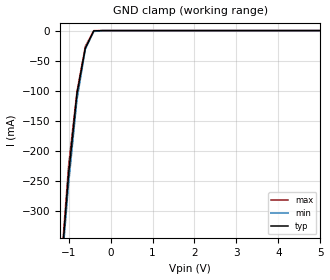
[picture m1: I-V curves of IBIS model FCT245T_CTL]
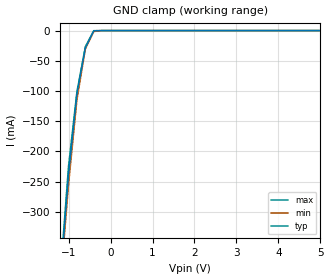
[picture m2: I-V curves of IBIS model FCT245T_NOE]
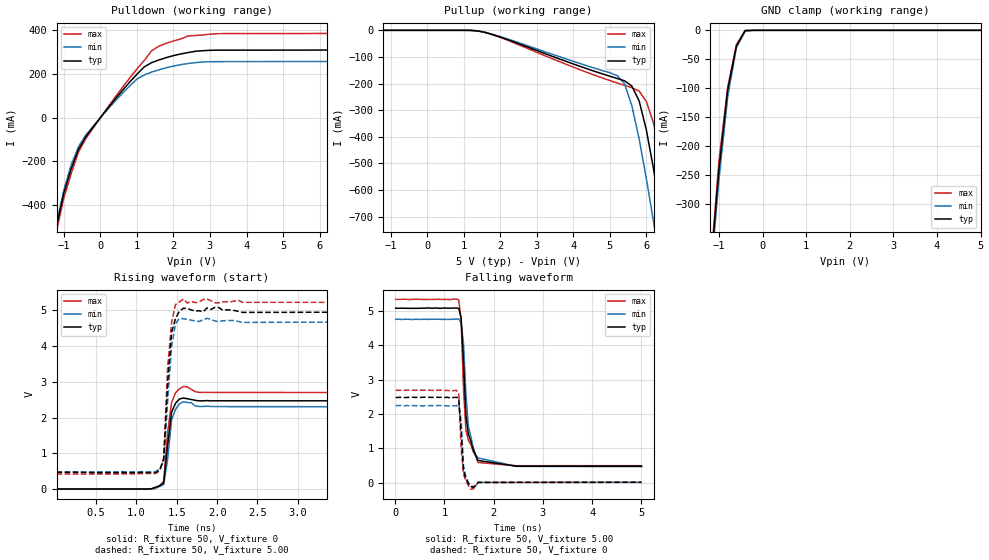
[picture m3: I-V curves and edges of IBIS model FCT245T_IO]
|   TEXAS INSTRUMENTS INCORPORATED
|   Standard Linear and Logic
|   IBIS Model of CY74FCT245T
|   8-BIT TRANSCEIVERS WITH 3-STATE OUTPUTS
|   DIP 20-pin (P), QSOP 20-pin (Q), SOIC 20-pin (SO)
[IBIS Ver]   3.1
[Comment Char]  |_char
[File Name]   cy74fct245t.ibs
[File Rev]   1.1
[Date]   June 4, 2004
[Source]   File originated at Texas Instruments, Inc.
[Notes]   The following is a sample IBIS file for the FCT245T.
   - FILE REV HISTORY
   - 1.1 Release IBIS file on 06/08/04
   - All test data contained in this file are derived from
   actual measurements.
   - Power clamp data deleted as there is no power-clamp diode.
   - The measurement used P package.
[Disclaimer] Property of Texas Instruments Incorporated.  Unauthorized
   reproduction and/or distribution is strictly prohibited.
   This product is protected under copyright law.
   Created 2000, (C) Copyright 2000, Texas Instruments Inc.,
   All Rights Reserved.
   UNLESS THERE IS A SIGNED, WRITTEN AGREEMENT TO THE
   CONTRARY, TEXAS INSTRUMENTS () IS PROVIDING THE IBIS
   MODELS  AND WITHOUT ANY WARRANTY, EXPRESSED OR
   IMPLIED.  TI assumes no liability for:
   1) the accuracy of the IBIS models provided to your
   company;
   2) the proper functioning of these IBIS Models in your
   design or for any resulting applications; or
   3) infringement of patents, copyrights or intellectual
   property rights resulting from your use of these IBIS
   models.
   TI provides IBIS Models as a service to our customers.
   You and your company shall not distribute, sell or give
   these models to anyone else without prior written
   permission from TI.
   TI reserves the right to make changes to our products or
   to discontinue any semiconductor product or service
   without notice, and advises our customers to obtain the
   latest version of relevant information to verify, before
   placing orders, that the information being relied on is
   current.
   Please be aware that your receipt and use of the IBIS
   information provided shall serve as acceptance of these
   terms and conditions.  If you do not accept these terms,
   you should return or destroy the IBIS models and any
   other accompanying information immediately.
|   Component FCT245T_P
[Component]   FCT245T_P
[Manufacturer]  Texas Instruments, Inc.
[Package]
|   typ   min   max
R_pkg   0.043   0.038   0.05
L_pkg   7.384nH   4.68nH   10.321nH
C_pkg   0.510pF   0.231pF   0.821pF
[Pin]   signal_name   model_name   R_pin   L_pin   C_pin
1   T/NR   FCT245T_CTL   0.042   9.427nH   0.81pF
2   A0   FCT245T_IO   0.046   8.544nH   0.456pF
3   A1   FCT245T_IO   0.048   7.163nH   0.435pF
4   A2   FCT245T_IO   0.040   4.825nH   0.261pF
5   A3   FCT245T_IO   0.040   5.284nH   0.648pF
6   A4   FCT245T_IO   0.040   4.686nH   0.232pF
7   A5   FCT245T_IO   0.040   6.359nH   0.489pF
8   A6   FCT245T_IO   0.038   7.982nH   0.475pF
9   A7   FCT245T_IO   0.043   9.403nH   0.475pF
10   GND   GND   0.050   10.321nH   0.805pF
11   B0   FCT245T_IO   0.050   10.281nH   0.810pF
12   B1   FCT245T_IO   0.043   9.383nH   0.477pF
13   B2   FCT245T_IO   0.038   7.978nH   0.476pF
14   B3   FCT245T_IO   0.040   6.302nH   0.492pF
15   B4   FCT245T_IO   0.040   4.680nH   0.231pF
16   B5   FCT245T_IO   0.040   5.284nH   0.648pF
17   B6   FCT245T_IO   0.040   4.822nH   0.261pF
18   B7   FCT245T_IO   0.047   7.118nH   0.439pF
19   NOE   FCT245T_NOE   0.046   8.492nH   0.461pF
20   VCC   POWER   0.043   9.348nH   0.821pF
|   Component FCT245T_Q
[Component]   FCT245T_Q
[Manufacturer]  Texas Instruments, Inc.
[Package]
|   typ   min   max
R_pkg   0.044   0.029   0.058
L_pkg   3.666nH   2.317nH   5.115nH
C_pkg   0.548pF   0.316pF   0.725pF
[Pin]   signal_name   model_name   R_pin   L_pin   C_pin
1   T/NR   FCT245T_CTL   0.058   5.115nH   0.725pF
2   A0   FCT245T_IO   0.053   4.591nH   0.724pF
3   A1   FCT245T_IO   0.049   3.754nH   0.572pF
4   A2   FCT245T_IO   0.029   2.549nH   0.388pF
5   A3   FCT245T_IO   0.031   2.317nH   0.316pF
6   A4   FCT245T_IO   0.031   2.317nH   0.316pF
7   A5   FCT245T_IO   0.029   2.556nH   0.399pF
8   A6   FCT245T_IO   0.049   3.754nH   0.579pF
9   A7   FCT245T_IO   0.053   4.591nH   0.724pF
10   GND   GND   0.058   5.115nH   0.725pF
11   B0   FCT245T_IO   0.058   5.115nH   0.725pF
12   B1   FCT245T_IO   0.053   4.591nH   0.724pF
13   B2   FCT245T_IO   0.049   3.754nH   0.579pF
14   B3   FCT245T_IO   0.029   2.557nH   0.399pF
15   B4   FCT245T_IO   0.031   2.317nH   0.316pF
16   B5   FCT245T_IO   0.031   2.317nH   0.316pF
17   B6   FCT245T_IO   0.029   2.557nH   0.399pF
18   B7   FCT245T_IO   0.049   3.754nH   0.579pF
19   NOE   FCT245T_NOE   0.053   4.591nH   0.724pF
20   VCC   POWER   0.058   5.115nH   0.725pF
|   Component FCT245T_SO
[Component]   FCT245T_SO
[Manufacturer]  Texas Instruments, Inc.
[Package]
|   typ   min   max
R_pkg   0.044   0.029   0.058
L_pkg   3.666nH   2.317nH   5.115nH
C_pkg   0.548pF   0.316pF   0.725pF
[Pin]   signal_name   model_name   R_pin   L_pin   C_pin
1   T/NR   FCT245T_CTL   0.058   5.115nH   0.725pF
2   A0   FCT245T_IO   0.053   4.591nH   0.724pF
3   A1   FCT245T_IO   0.049   3.754nH   0.572pF
4   A2   FCT245T_IO   0.029   2.549nH   0.388pF
5   A3   FCT245T_IO   0.031   2.317nH   0.316pF
6   A4   FCT245T_IO   0.031   2.317nH   0.316pF
7   A5   FCT245T_IO   0.029   2.556nH   0.399pF
8   A6   FCT245T_IO   0.049   3.754nH   0.579pF
9   A7   FCT245T_IO   0.053   4.591nH   0.724pF
10   GND   GND   0.058   5.115nH   0.725pF
11   B0   FCT245T_IO   0.058   5.115nH   0.725pF
12   B1   FCT245T_IO   0.053   4.591nH   0.724pF
13   B2   FCT245T_IO   0.049   3.754nH   0.579pF
14   B3   FCT245T_IO   0.029   2.557nH   0.399pF
15   B4   FCT245T_IO   0.031   2.317nH   0.316pF
16   B5   FCT245T_IO   0.031   2.317nH   0.316pF
17   B6   FCT245T_IO   0.029   2.557nH   0.399pF
18   B7   FCT245T_IO   0.049   3.754nH   0.579pF
19   NOE   FCT245T_NOE   0.053   4.591nH   0.724pF
20   VCC   POWER   0.058   5.115nH   0.725pF
| Models and submodels in the file (3): FCT245T_CTL (Input), FCT245T_NOE (Input), FCT245T_IO (I/O)
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|   Model FCT245T_CTL
[Model]   FCT245T_CTL
Model_type  Input
Polarity   Inverting
Vinl = 0.8
Vinh = 2.0
| variable   typ   min   max
C_comp   7.394pf   6.096pF   9.010pf
[Temperature Range]   25   85   -40
[Voltage Range]   5.00   4.75   5.25
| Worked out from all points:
|   GND clamp passes 1 mA (typ) near -0.40 V on its own axis
[GND Clamp]
|   Voltage   I(typ)   I(min)   I(max)
-5V       -4.468A    -4.116A    -4.74A
-1.2V     -416.2mA   -425.6mA   -409.2mA
-1V       -238.8mA   -255.3mA   -224.6mA
-800mV    -104.8mA   -115.1mA   -101.1mA
-600mV    -28.96mA   -30.97mA   -26mA
-400mV    -505.9uA   -1.622mA   -97.14uA
-200mV    -1.141uA   -7.754uA   -501nA
5V        765pA      14.39nA    212.3nA
|   Model FCT245T_NOE
[Model]   FCT245T_NOE
Model_type  Input
Polarity   Inverting
Vinl = 0.8
Vinh = 2.0
| variable   typ   min   max
C_comp   7.364pf   6.038pF   9.040pf
[Temperature Range]   25   85   -40
[Voltage Range]   5.00   4.75   5.25
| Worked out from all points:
|   GND clamp passes 1 mA (typ) near -0.40 V on its own axis
[GND Clamp]
|   Voltage   I(typ)   I(min)   I(max)
-5V       -4.466A    -4.125A    -4.736A
-1.2V     -416mA     -425.7mA   -408.3mA
-1V       -238.3mA   -254.7mA   -224.2mA
-800mV    -104.5mA   -114.3mA   -101mA
-600mV    -28.77mA   -30.58mA   -26.7mA
-400mV    -490.6uA   -1.585mA   -105.2uA
-200mV    -946nA     -6.848uA   -3.231uA
5V        526.4pA    12.23nA    261.7nA
|   Model FCT245T_IO
[Model]   FCT245T_IO
Model_type  I/O
Polarity   Non-Inverting
Enable   Active-Low
Vmeas = 1.5v
Cref = 50pf
Vinl = 0.8
Vinh = 2.0
| variable   typ   min   max
C_comp   6.618pF   5.970pF   7.170pF
[Temperature Range]   25   85   -40
[Voltage Range]   5.00   4.75   5.25
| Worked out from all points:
|   slope of the pulldown table from 0 to 0.75 V, typ, clamps not added: 4.9 ohm
|   GND clamp passes 1 mA (typ) near -0.40 V on its own axis
|   rising waveform, R_fixture 50, V_fixture 0: 20-80 % time 73.6ps typ, 70.6ps min, 71.1ps max; typ from 0.005 V to 2.47 V
|   falling waveform, R_fixture 50, V_fixture 5.00: 20-80 % time 127ps typ, 145ps min, 98.9ps max; typ from 5.08 V to 0.472 V
|   rising waveform, R_fixture 50, V_fixture 5.00: 20-80 % time 74.4ps typ, 77.4ps min, 72.6ps max; typ from 0.465 V to 4.95 V
|   falling waveform, R_fixture 50, V_fixture 0: 20-80 % time 66.5ps typ, 52.5ps min, 64.5ps max; typ from 2.48 V to 0.008 V
[Pulldown]
|   Voltage   I(typ)   I(min)   I(max)
-5V       -4.144A    -3.944A    -4.446A
-1.2V     -496mA     -483.4mA   -517.7mA
-1V       -344.7mA   -332mA     -367mA
-800mV    -234mA     -216.1mA   -255.9mA
-600mV    -145.3mA   -132.9mA   -156.9mA
-400mV    -87.36mA   -79.07mA   -96.07mA
1V        198.8mA    176.6mA    222.9mA
1.4V      251.9mA    208.7mA    305.9mA
1.8V      274.9mA    228.5mA    340.2mA
3.2V      309.2mA    256.6mA    384.4mA
6.6V      310.1mA    259.2mA    385.7mA
10V       346.5mA    280.6mA    415.3mA
[Pullup]
|   Voltage   I(typ)   I(min)   I(max)
-5V       13.94nA    95.06nA    6.632uA
1.4V      -2.646mA   -3.207mA   -1.9mA
5V        -172.6mA   -159.6mA   -188.8mA
5.4V      -189.6mA   -200.6mA   -206.9mA
5.6V      -209.7mA   -283mA     -215.5mA
5.8V      -265mA     -408.2mA   -228.3mA
6V        -375.8mA   -559.8mA   -268.3mA
6.2V      -525.6mA   -724.9mA   -351.4mA
6.4V      -699mA     -890.1mA   -492.3mA
6.6V      -883mA     -1.055A    -669.7mA
6.8V      -1.067A    -1.22A     -866.2mA
10V       -4.004A    -3.864A    -4.038A
[GND Clamp]
|   Voltage   I(typ)   I(min)   I(max)
-5V       -4.495A    -4.147A    -4.786A
-1.2V     -420.1mA   -430.1mA   -411.8mA
-1V       -239.7mA   -257.2mA   -224.7mA
-800mV    -102.9mA   -114.5mA   -97.89mA
-600mV    -27.08mA   -29.63mA   -24.52mA
-400mV    -485.1uA   -1.539mA   -106.4uA
-200mV    -1.891uA   -8.632uA   -5.169uA
5V        2.72nA     30.82nA    -46.98nA
[Ramp]
| variable   typ   min   max
dV/dt_r  1.362E+00/5.600E-10  1.344E+00/5.840E-10  1.620E+00/5.070E-10
dV/dt_f  2.790E+00/1.145E-09  2.658E+00/1.389E-09  2.944E+00/9.350E-10
R_load = 50
[Rising Waveform]
R_fixture = 50
V_fixture = 0
V_fixture_min = 0
V_fixture_max = 0
C_fixture = 0pf
L_fixture = 0nH
|   Time   V(typ)   V(min)   V(max)
9.766ps   4.889mV    8.362mV    82.4uV
1.182ns   9.065mV    8.076mV    1.114mV
1.289ns   94.61mV    78.28mV    103.9mV
1.338ns   173.2mV    131.4mV    221.1mV
1.387ns   1.24V      845.5mV    1.598V
1.436ns   2.152V     1.939V     2.423V
1.484ns   2.401V     2.229V     2.695V
1.582ns   2.547V     2.442V     2.869V
1.777ns   2.468V     2.312V     2.704V
5ns       2.469V     2.3V       2.701V
[Falling Waveform]
R_fixture = 50
V_fixture = 5.00
V_fixture_min = 4.75
V_fixture_max = 5.25
C_fixture = 0pf
L_fixture = 0nH
|   Time   V(typ)   V(min)   V(max)
9.766ps   5.077V     4.752V     5.335V
1.289ns   5.074V     4.762V     5.319V
1.338ns   4.807V     4.651V     4.733V
1.387ns   3.496V     4.048V     2.722V
1.436ns   1.964V     2.565V     1.516V
1.484ns   1.415V     1.643V     1.239V
1.582ns   955.7mV    1.03V      908mV
1.68ns    643.6mV    717.4mV    583.9mV
2.461ns   475mV      470.2mV    489.6mV
5ns       472.2mV    466.9mV    490.1mV
[Rising Waveform]
R_fixture = 50
V_fixture = 5.00
V_fixture_min = 4.75
V_fixture_max = 5.25
C_fixture = 0pf
L_fixture = 0nH
|   Time   V(typ)   V(min)   V(max)
9.766ps   465.3mV    482.6mV    421.6mV
1.289ns   534.4mV    583.4mV    518.7mV
1.338ns   829.3mV    784.9mV    863.4mV
1.387ns   2.976V     2.47V      3.409V
1.436ns   4.384V     3.996V     4.656V
1.484ns   4.765V     4.627V     5.161V
1.582ns   5.057V     4.762V     5.311V
1.631ns   5.05V      4.746V     5.204V
1.875ns   5.066V     4.775V     5.314V
5ns       4.953V     4.681V     5.224V
[Falling Waveform]
R_fixture = 50
V_fixture = 0
V_fixture_min = 0
V_fixture_max = 0
C_fixture = 0pf
L_fixture = 0nH
|   Time   V(typ)   V(min)   V(max)
9.766ps   2.475V     2.239V     2.688V
1.24ns    2.482V     2.24V      2.685V
1.289ns   2.466V     2.24V      2.616V
1.338ns   1.493V     1.826V     1.002V
1.387ns   333.1mV    484.6mV    244.8mV
1.436ns   119.9mV    163.6mV    42.27mV
1.533ns   -118.7mV   -85.6mV    -192.9mV
1.631ns   -91.55mV   -97.35mV   -116.3mV
1.68ns    3.826mV    3.311mV    4.388mV
5ns       7.715mV    7.263mV    8.301mV
